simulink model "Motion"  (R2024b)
settings: Solver=VariableStepAuto  StartTime=0.0  StopTime=10.0  RelTol=1e-3
undefined symbols (not defined in the file): deg, kg, m, N, s, X, Y, Z
libraries: sm_lib x12, nesl_utility x2, SignalEditorBlockLib x1

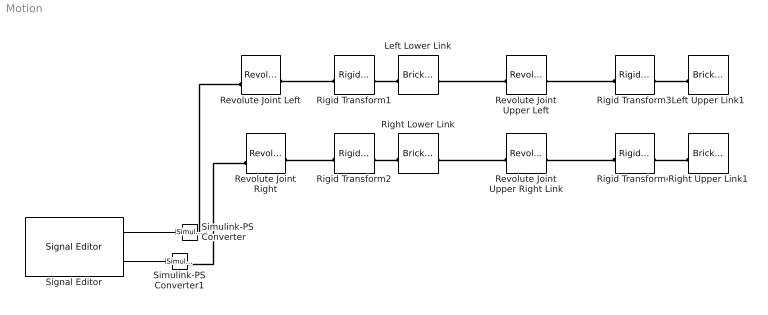
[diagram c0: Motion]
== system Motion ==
  Left Lower Link : sm_lib/Body Elements/Brick Solid  BrickDimensions=[2 12 0.5]  BrickDimensionsUnits=cm  ExportEntireGeometry=off  InertiaType=CalculateFromGeometry  BasedOnType=Density  Density=1000  DensityUnits=kg/m^3  Mass=1  MassUnits=kg  CenterOfMass=[0 0 0]  CenterOfMassUnits=m  MomentsOfInertia=[1 1 1]  MomentsOfInertiaUnits=kg*m^2  ProductsOfInertia=[0 0 0]  ProductsOfInertiaUnits=kg*m^2  GraphicType=FromGeometry  MarkerShape=Sphere  MarkerSize=10  GraphicVisPropType=SimpleVisualProperties  GraphicDiffuseColor=[0.5 0.5 0.5]  GraphicOpacity=1  GraphicSpecularColor=[0.5 0.5 0.5 1.0]  GraphicAmbientColor=[0.15 0.15 0.15 1.0]  GraphicEmissiveColor=[0.0 0.0 0.0 1.0]  GraphicShininess=75  DoExposeReferenceFrame=on  SerializedFrames=<Frames><Frame><Id>Frame1</Id><Value><Name>F1</Name><Origin><Source>ReferenceFrame</Source><FeatureName></FeatureName></Origin><PrimaryAxis><DefinedDirection>+Z</DefinedDirection><Source>ReferenceFrame</Source><SourceDirection>+Z</SourceDirection><FeatureName></FeatureName></PrimaryAxis><SecondaryAxis><DefinedDirection>+X</DefinedDirection><Source>ReferenceFrame</Source><SourceDirection>+X</Source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
  Left Upper Link1 : sm_lib/Body Elements/Brick Solid  BrickDimensions=[2 12 0.5]  BrickDimensionsUnits=cm  ExportEntireGeometry=off  InertiaType=CalculateFromGeometry  BasedOnType=Density  Density=1000  DensityUnits=kg/m^3  Mass=1  MassUnits=kg  CenterOfMass=[0 0 0]  CenterOfMassUnits=m  MomentsOfInertia=[1 1 1]  MomentsOfInertiaUnits=kg*m^2  ProductsOfInertia=[0 0 0]  ProductsOfInertiaUnits=kg*m^2  GraphicType=FromGeometry  MarkerShape=Sphere  MarkerSize=10  GraphicVisPropType=SimpleVisualProperties  GraphicDiffuseColor=[0.5 0.5 0.5]  GraphicOpacity=1  GraphicSpecularColor=[0.5 0.5 0.5 1.0]  GraphicAmbientColor=[0.15 0.15 0.15 1.0]  GraphicEmissiveColor=[0.0 0.0 0.0 1.0]  GraphicShininess=75  DoExposeReferenceFrame=on  SerializedFrames=<Frames><Frame><Id>Frame1</Id><Value><Name>F1</Name><Origin><Source>ReferenceFrame</Source><FeatureName></FeatureName></Origin><PrimaryAxis><DefinedDirection>+Z</DefinedDirection><Source>ReferenceFrame</Source><SourceDirection>+Z</SourceDirection><FeatureName></FeatureName></PrimaryAxis><SecondaryAxis><DefinedDirection>+X</DefinedDirection><Source>ReferenceFrame</Source><SourceDirection>+X</Source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
  Revolute Joint Left : sm_lib/Joints/Revolute Joint  JointMode=Normal  CompositeWrenchDir=FollowerOnBase  CompositeWrenchFrame=BaseFrame  SenseConstraintForce=off  SenseConstraintTorque=off  SenseTotalForce=off  SenseTotalTorque=off  PositionTargetSpecify=off  PositionTargetPriority=High  PositionTargetValue=0  PositionTargetValueUnits=deg  VelocityTargetSpecify=off  VelocityTargetPriority=High  VelocityTargetValue=0  VelocityTargetValueUnits=deg/s  EquilibriumPosition=0  EquilibriumPositionUnits=deg  SpringStiffness=0  SpringStiffnessUnits=N*m/deg  DampingCoefficient=0  DampingCoefficientUnits=N*m/(deg/s)  LowerLimitSpecify=off  LowerLimitBound=-90  LowerLimitBoundUnits=deg  LowerLimitStiffness=1e4  LowerLimitStiffnessUnits=N*m/deg  LowerLimitDamping=10  LowerLimitDampingUnits=N*m/(deg/s)  LowerLimitTransitionRegionWidth=0.1  LowerLimitTransitionRegionWidthUnits=deg  UpperLimitSpecify=off  UpperLimitBound=90  UpperLimitBoundUnits=deg  UpperLimitStiffness=1e4  UpperLimitStiffnessUnits=N*m/deg  UpperLimitDamping=10  UpperLimitDampingUnits=N*m/(deg/s)  UpperLimitTransitionRegionWidth=0.1  UpperLimitTransitionRegionWidthUnits=deg  TorqueActuationMode=ComputedTorque  MotionActuationMode=InputMotion  SensePosition=off  SenseVelocity=off  SenseAcceleration=off  SenseTorqueForce=off  SenseLowerLimitTorqueForce=off  SenseUpperLimitTorqueForce=off
  Revolute Joint Right : sm_lib/Joints/Revolute Joint  JointMode=Normal  CompositeWrenchDir=FollowerOnBase  CompositeWrenchFrame=BaseFrame  SenseConstraintForce=off  SenseConstraintTorque=off  SenseTotalForce=off  SenseTotalTorque=off  PositionTargetSpecify=off  PositionTargetPriority=High  PositionTargetValue=0  PositionTargetValueUnits=deg  VelocityTargetSpecify=off  VelocityTargetPriority=High  VelocityTargetValue=0  VelocityTargetValueUnits=deg/s  EquilibriumPosition=0  EquilibriumPositionUnits=deg  SpringStiffness=0  SpringStiffnessUnits=N*m/deg  DampingCoefficient=0  DampingCoefficientUnits=N*m/(deg/s)  LowerLimitSpecify=off  LowerLimitBound=-90  LowerLimitBoundUnits=deg  LowerLimitStiffness=1e4  LowerLimitStiffnessUnits=N*m/deg  LowerLimitDamping=10  LowerLimitDampingUnits=N*m/(deg/s)  LowerLimitTransitionRegionWidth=0.1  LowerLimitTransitionRegionWidthUnits=deg  UpperLimitSpecify=off  UpperLimitBound=90  UpperLimitBoundUnits=deg  UpperLimitStiffness=1e4  UpperLimitStiffnessUnits=N*m/deg  UpperLimitDamping=10  UpperLimitDampingUnits=N*m/(deg/s)  UpperLimitTransitionRegionWidth=0.1  UpperLimitTransitionRegionWidthUnits=deg  TorqueActuationMode=ComputedTorque  MotionActuationMode=InputMotion  SensePosition=off  SenseVelocity=off  SenseAcceleration=off  SenseTorqueForce=off  SenseLowerLimitTorqueForce=off  SenseUpperLimitTorqueForce=off
  Revolute Joint Upper Left : sm_lib/Joints/Revolute Joint  JointMode=Normal  CompositeWrenchDir=FollowerOnBase  CompositeWrenchFrame=BaseFrame  SenseConstraintForce=off  SenseConstraintTorque=off  SenseTotalForce=off  SenseTotalTorque=off  PositionTargetSpecify=off  PositionTargetPriority=High  PositionTargetValue=0  PositionTargetValueUnits=deg  VelocityTargetSpecify=off  VelocityTargetPriority=High  VelocityTargetValue=0  VelocityTargetValueUnits=deg/s  EquilibriumPosition=0  EquilibriumPositionUnits=deg  SpringStiffness=0  SpringStiffnessUnits=N*m/deg  DampingCoefficient=0  DampingCoefficientUnits=N*m/(deg/s)  LowerLimitSpecify=off  LowerLimitBound=-90  LowerLimitBoundUnits=deg  LowerLimitStiffness=1e4  LowerLimitStiffnessUnits=N*m/deg  LowerLimitDamping=10  LowerLimitDampingUnits=N*m/(deg/s)  LowerLimitTransitionRegionWidth=0.1  LowerLimitTransitionRegionWidthUnits=deg  UpperLimitSpecify=off  UpperLimitBound=90  UpperLimitBoundUnits=deg  UpperLimitStiffness=1e4  UpperLimitStiffnessUnits=N*m/deg  UpperLimitDamping=10  UpperLimitDampingUnits=N*m/(deg/s)  UpperLimitTransitionRegionWidth=0.1  UpperLimitTransitionRegionWidthUnits=deg  TorqueActuationMode=NoTorque  MotionActuationMode=ComputedMotion  SensePosition=off  SenseVelocity=off  SenseAcceleration=off  SenseTorqueForce=off  SenseLowerLimitTorqueForce=off  SenseUpperLimitTorqueForce=off
  Revolute Joint Upper Right Link : sm_lib/Joints/Revolute Joint  JointMode=Normal  CompositeWrenchDir=FollowerOnBase  CompositeWrenchFrame=BaseFrame  SenseConstraintForce=off  SenseConstraintTorque=off  SenseTotalForce=off  SenseTotalTorque=off  PositionTargetSpecify=off  PositionTargetPriority=High  PositionTargetValue=0  PositionTargetValueUnits=deg  VelocityTargetSpecify=off  VelocityTargetPriority=High  VelocityTargetValue=0  VelocityTargetValueUnits=deg/s  EquilibriumPosition=0  EquilibriumPositionUnits=deg  SpringStiffness=0  SpringStiffnessUnits=N*m/deg  DampingCoefficient=0  DampingCoefficientUnits=N*m/(deg/s)  LowerLimitSpecify=off  LowerLimitBound=-90  LowerLimitBoundUnits=deg  LowerLimitStiffness=1e4  LowerLimitStiffnessUnits=N*m/deg  LowerLimitDamping=10  LowerLimitDampingUnits=N*m/(deg/s)  LowerLimitTransitionRegionWidth=0.1  LowerLimitTransitionRegionWidthUnits=deg  UpperLimitSpecify=off  UpperLimitBound=90  UpperLimitBoundUnits=deg  UpperLimitStiffness=1e4  UpperLimitStiffnessUnits=N*m/deg  UpperLimitDamping=10  UpperLimitDampingUnits=N*m/(deg/s)  UpperLimitTransitionRegionWidth=0.1  UpperLimitTransitionRegionWidthUnits=deg  TorqueActuationMode=NoTorque  MotionActuationMode=ComputedMotion  SensePosition=off  SenseVelocity=off  SenseAcceleration=off  SenseTorqueForce=off  SenseLowerLimitTorqueForce=off  SenseUpperLimitTorqueForce=off
  Right Lower Link : sm_lib/Body Elements/Brick Solid  BrickDimensions=[2 12 0.5]  BrickDimensionsUnits=cm  ExportEntireGeometry=off  InertiaType=CalculateFromGeometry  BasedOnType=Density  Density=1000  DensityUnits=kg/m^3  Mass=1  MassUnits=kg  CenterOfMass=[0 0 0]  CenterOfMassUnits=m  MomentsOfInertia=[1 1 1]  MomentsOfInertiaUnits=kg*m^2  ProductsOfInertia=[0 0 0]  ProductsOfInertiaUnits=kg*m^2  GraphicType=FromGeometry  MarkerShape=Sphere  MarkerSize=10  GraphicVisPropType=SimpleVisualProperties  GraphicDiffuseColor=[0.5 0.5 0.5]  GraphicOpacity=1  GraphicSpecularColor=[0.5 0.5 0.5 1.0]  GraphicAmbientColor=[0.15 0.15 0.15 1.0]  GraphicEmissiveColor=[0.0 0.0 0.0 1.0]  GraphicShininess=75  DoExposeReferenceFrame=on  SerializedFrames=<Frames><Frame><Id>Frame1</Id><Value><Name>F1</Name><Origin><Source>ReferenceFrame</Source><FeatureName></FeatureName></Origin><PrimaryAxis><DefinedDirection>+Z</DefinedDirection><Source>ReferenceFrame</Source><SourceDirection>+Z</SourceDirection><FeatureName></FeatureName></PrimaryAxis><SecondaryAxis><DefinedDirection>+X</DefinedDirection><Source>ReferenceFrame</Source><SourceDirection>+X</Source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
  Right Upper Link1 : sm_lib/Body Elements/Brick Solid  BrickDimensions=[2 12 0.5]  BrickDimensionsUnits=cm  ExportEntireGeometry=off  InertiaType=CalculateFromGeometry  BasedOnType=Density  Density=1000  DensityUnits=kg/m^3  Mass=1  MassUnits=kg  CenterOfMass=[0 0 0]  CenterOfMassUnits=m  MomentsOfInertia=[1 1 1]  MomentsOfInertiaUnits=kg*m^2  ProductsOfInertia=[0 0 0]  ProductsOfInertiaUnits=kg*m^2  GraphicType=FromGeometry  MarkerShape=Sphere  MarkerSize=10  GraphicVisPropType=SimpleVisualProperties  GraphicDiffuseColor=[0.5 0.5 0.5]  GraphicOpacity=1  GraphicSpecularColor=[0.5 0.5 0.5 1.0]  GraphicAmbientColor=[0.15 0.15 0.15 1.0]  GraphicEmissiveColor=[0.0 0.0 0.0 1.0]  GraphicShininess=75  DoExposeReferenceFrame=on  SerializedFrames=<Frames><Frame><Id>Frame1</Id><Value><Name>F1</Name><Origin><Source>ReferenceFrame</Source><FeatureName></FeatureName></Origin><PrimaryAxis><DefinedDirection>+Z</DefinedDirection><Source>ReferenceFrame</Source><SourceDirection>+Z</SourceDirection><FeatureName></FeatureName></PrimaryAxis><SecondaryAxis><DefinedDirection>+X</DefinedDirection><Source>ReferenceFrame</Source><SourceDirection>+X</Source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
  Rigid Transform1 : sm_lib/Frames and Transforms/Rigid Transform  RotationMethod=StandardAxis  FollAlignAxisA=+X  BaseAlignAxisA=+Y  FollAlignAxisB=+Y  BaseAlignAxisB=+Z  RotationStandardAxis=+Z  RotationAngle=30  RotationAngleUnits=deg  RotationArbitraryAxis=[0 0 1]  RotationSequenceAxes=FollowerAxes  RotationSequence=XYX  RotationSequenceAngles=[0 0 0]  RotationSequenceAnglesUnits=deg  RotationMatrix=[1 0 0;0 1 0;0 0 1]  Quaternion=[1 0 0 0]  TranslationMethod=Cartesian  TranslationCartesianOffset=[-1 5 3]  TranslationCartesianOffsetUnits=cm  TranslationStandardAxis=+Z  TranslationStandardOffset=0  TranslationStandardOffsetUnits=m  TranslationROffset=0  TranslationROffsetUnits=m  TranslationThetaOffset=0  TranslationThetaOffsetUnits=deg  TranslationZOffset=0  TranslationZOffsetUnits=m
  Rigid Transform2 : sm_lib/Frames and Transforms/Rigid Transform  RotationMethod=StandardAxis  FollAlignAxisA=+X  BaseAlignAxisA=+Y  FollAlignAxisB=+Y  BaseAlignAxisB=+Z  RotationStandardAxis=+Z  RotationAngle=-30  RotationAngleUnits=deg  RotationArbitraryAxis=[0 0 1]  RotationSequenceAxes=FollowerAxes  RotationSequence=XYX  RotationSequenceAngles=[0 0 0]  RotationSequenceAnglesUnits=deg  RotationMatrix=[1 0 0;0 1 0;0 0 1]  Quaternion=[1 0 0 0]  TranslationMethod=Cartesian  TranslationCartesianOffset=[-1 -5 3]  TranslationCartesianOffsetUnits=cm  TranslationStandardAxis=+Z  TranslationStandardOffset=0  TranslationStandardOffsetUnits=m  TranslationROffset=0  TranslationROffsetUnits=m  TranslationThetaOffset=0  TranslationThetaOffsetUnits=deg  TranslationZOffset=0  TranslationZOffsetUnits=m
  Rigid Transform3 : sm_lib/Frames and Transforms/Rigid Transform  RotationMethod=StandardAxis  FollAlignAxisA=+X  BaseAlignAxisA=+Y  FollAlignAxisB=+Y  BaseAlignAxisB=+Z  RotationStandardAxis=+Z  RotationAngle=-75  RotationAngleUnits=deg  RotationArbitraryAxis=[0 0 1]  RotationSequenceAxes=FollowerAxes  RotationSequence=XYX  RotationSequenceAngles=[0 0 0]  RotationSequenceAnglesUnits=deg  RotationMatrix=[1 0 0;0 1 0;0 0 1]  Quaternion=[1 0 0 0]  TranslationMethod=Cartesian  TranslationCartesianOffset=[4.8 7 0.6]  TranslationCartesianOffsetUnits=cm  TranslationStandardAxis=+Z  TranslationStandardOffset=0  TranslationStandardOffsetUnits=m  TranslationROffset=0  TranslationROffsetUnits=m  TranslationThetaOffset=0  TranslationThetaOffsetUnits=deg  TranslationZOffset=0  TranslationZOffsetUnits=m
  Rigid Transform4 : sm_lib/Frames and Transforms/Rigid Transform  RotationMethod=StandardAxis  FollAlignAxisA=+X  BaseAlignAxisA=+Y  FollAlignAxisB=+Y  BaseAlignAxisB=+Z  RotationStandardAxis=+Z  RotationAngle=75  RotationAngleUnits=deg  RotationArbitraryAxis=[0 0 1]  RotationSequenceAxes=FollowerAxes  RotationSequence=XYX  RotationSequenceAngles=[0 0 0]  RotationSequenceAnglesUnits=deg  RotationMatrix=[1 0 0;0 1 0;0 0 1]  Quaternion=[1 0 0 0]  TranslationMethod=Cartesian  TranslationCartesianOffset=[4.8 -7 0.6]  TranslationCartesianOffsetUnits=cm  TranslationStandardAxis=+Z  TranslationStandardOffset=0  TranslationStandardOffsetUnits=m  TranslationROffset=0  TranslationROffsetUnits=m  TranslationThetaOffset=0  TranslationThetaOffsetUnits=deg  TranslationZOffset=0  TranslationZOffsetUnits=m
  Signal Editor : SignalEditorBlockLib/Signal Editor  FileName=/MATLAB Drive/Robotic Arm/LeftJointSignal.mat  ActiveScenario=Scenario  ActiveSignal=Left Joint  IsBus=off  OutputBusObjectStr=Bus: BusObject  SampleTime=0  ZeroCross=off  OutputAfterFinalValue=Setting to zero  Unit=deg  PreserveSignalName=on  ApplySigPropsToAllScenarios=on  ApplySigPropsToAllSignals=on
  Simulink-PS Converter : nesl_utility/Simulink-PS Converter  PhysicalDomain=network_engine_domain  SubClassName=ps_input  LeftPortType=input  RightPortType=output  PseudoPeriodic=off  Frequencies=[]  NoiseDistribution=none  NoiseParameters=[]  Unit=rad  AffineConversion=off  FilteringAndDerivatives=zero  SimscapeFilterOrder=1  InputFilterTimeConstant=0.001  UdotUserProvided=0
  Simulink-PS Converter1 : nesl_utility/Simulink-PS Converter  PhysicalDomain=network_engine_domain  SubClassName=ps_input  LeftPortType=input  RightPortType=output  PseudoPeriodic=off  Frequencies=[]  NoiseDistribution=none  NoiseParameters=[]  Unit=rad  AffineConversion=off  FilteringAndDerivatives=zero  SimscapeFilterOrder=1  InputFilterTimeConstant=0.001  UdotUserProvided=0
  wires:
  Signal Editor/2 -> Simulink-PS Converter1/1
  Signal Editor/1 -> Simulink-PS Converter/1
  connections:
  Simulink-PS Converter/RConn1 -- Revolute Joint Left/LConn2
  Revolute Joint Right/RConn1 -- Rigid Transform2/LConn1
  Revolute Joint Upper Left/LConn1 -- Left Lower Link/RConn1
  Simulink-PS Converter1/RConn1 -- Revolute Joint Right/LConn2
  Rigid Transform2/RConn1 -- Right Lower Link/LConn1
  Revolute Joint Left/RConn1 -- Rigid Transform1/LConn1
  Rigid Transform3/RConn1 -- Left Upper Link1/LConn1
  Rigid Transform4/RConn1 -- Right Upper Link1/LConn1
  Revolute Joint Upper Right Link/RConn1 -- Rigid Transform4/LConn1
  Revolute Joint Upper Left/RConn1 -- Rigid Transform3/LConn1
  Revolute Joint Upper Right Link/LConn1 -- Right Lower Link/RConn1
  Rigid Transform1/RConn1 -- Left Lower Link/LConn1
